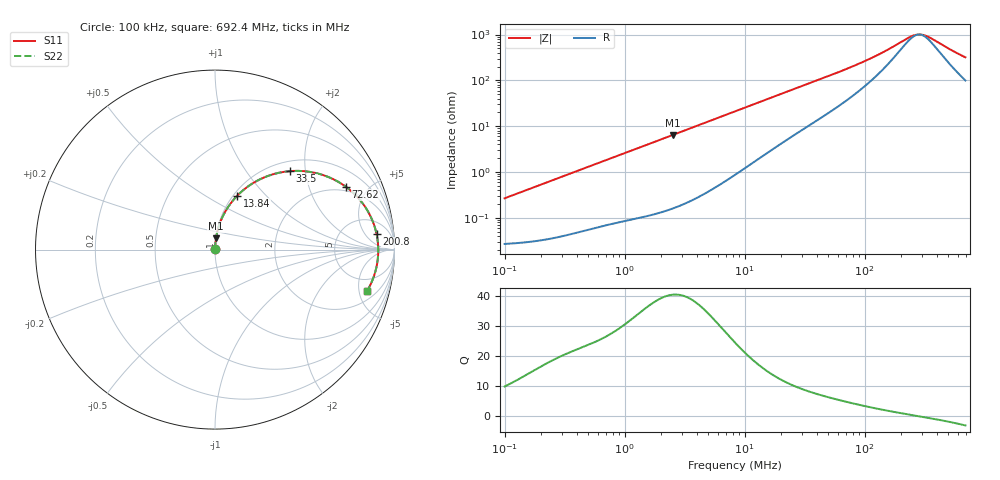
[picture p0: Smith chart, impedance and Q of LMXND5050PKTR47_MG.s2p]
! LMXND5050PKTR47_MG  S-PARAMETER MODEL  ( General Type )
! Model Generated by TAIYO YUDEN Corporation (https://www.yuden.co.jp/en/)
! Version 1.0
! TAIYO YUDEN Control No. 191023NI43SB-FBB
! Copyright(c) 2019 TAIYO YUDEN CO.,LTD. All Rights Reserved.
! Product Description (link to TY-COMPAS)
! https://ds.yuden.co.jp/TYCOMPAS/or/detail?pn=LMXND5050PKTR47NMG&u=M
! Products Name : Inductors
! Characteristics :
!  Inductance : 0.47 uH , SRF(min) : 185 MHz , DC Resistance(max) : 0.03 Ohm
!  Rated Current : Saturation :5800 mA , Temp Rise : 3300 mA (40 degC)
!  Case Size : 4.9 x 4.9 / 0.193 x 0.193 [mm/inch] , Thickness : 1.4 / 0.055 [mm/inch]
!  (Conditions: Temperature = 25 degC , DC Bias Current/Voltage = 0A / 0V)
! External Node Assignments :
!  1  o---GGG---o  2
! GND o---------o GND
! Frequency Range : 0.1MHz  -  692.442054MHz  [ 402 STEP ]
# MHz S RI R 50
! Freq[MHz].  S11 Real  S11 Imag  S21 Real  S21 Imag  S12 Real  S12 Imag  S22 Real  S22 Imag
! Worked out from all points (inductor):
!   401 points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, 100 kHz to 692.4 MHz, reference 50 ohm
!   read as one part in series: L = 423 nH near 104.5 kHz
!   highest Q = 40.3 at 2.522 MHz (marker M1), where L = 407 nH
!   self-resonance near 284.8 MHz
!   S11 on the Smith chart (normalised r, x): 100 kHz: 1.00, +0.01; 13.84 MHz: 1.04, +0.70; 33.5 MHz: 1.20, +1.65; 72.62 MHz: 1.77, +3.58; 200.8 MHz: 11, +10; 692.4 MHz: 2.99, -6.05
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0.1  0.000276 0.00266  0.9997 -0.00266  0.9997 -0.00266  0.000276 0.00266
0.439809  0.000638 0.0115  0.9994 -0.0115  0.9994 -0.0115  0.000638 0.0115
1.934321  0.00371 0.0492  0.9963 -0.0492  0.9963 -0.0492  0.00371 0.0492
2.52197  0.00571 0.064  0.9943 -0.064  0.9943 -0.064  0.00571 0.064
4.78815  0.018 0.1194  0.982 -0.1194  0.982 -0.1194  0.018 0.1194
8.507318  0.0524 0.2029  0.9476 -0.2029  0.9476 -0.2029  0.0524 0.2029
13.8361  0.1234 0.2997  0.8766 -0.2997  0.8766 -0.2997  0.1234 0.2997
21.05872  0.2368 0.3846  0.7632 -0.3846  0.7632 -0.3846  0.2368 0.3846
33.50056  0.4189 0.4373  0.5811 -0.4373  0.5811 -0.4373  0.4189 0.4373
36.59788  0.4574 0.4387  0.5426 -0.4387  0.5426 -0.4387  0.4574 0.4387
50.98828  0.6002 0.416  0.3998 -0.416  0.3998 -0.416  0.6002 0.416
72.62492  0.7298 0.3497  0.2702 -0.3497  0.2702 -0.3497  0.7298 0.3497
110.536  0.8339 0.242  0.1661 -0.242  0.1661 -0.242  0.8339 0.242
160.9608  0.8845 0.1422  0.1155 -0.1422  0.1155 -0.1422  0.8845 0.1422
200.7843  0.9003 0.086  0.0997 -0.086  0.0997 -0.086  0.9003 0.086
234.3886  0.9066 0.0476  0.0934 -0.0476  0.0934 -0.0476  0.9066 0.0476
256.0591  0.9086 0.026  0.0914 -0.026  0.0914 -0.026  0.9086 0.026
279.7333  0.9095 0.00437  0.0905 -0.00437  0.0905 -0.00437  0.9095 0.00437
305.5962  0.9094 -0.0172  0.0906 0.0172  0.0906 0.0172  0.9094 -0.0172
348.9424  0.9072 -0.0498  0.0928 0.0498  0.0928 0.0498  0.9072 -0.0498
531.0947  0.8822 -0.1575  0.1178 0.1575  0.1178 0.1575  0.8822 -0.1575
692.4421  0.8479 -0.2303  0.1521 0.2303  0.1521 0.2303  0.8479 -0.2303
